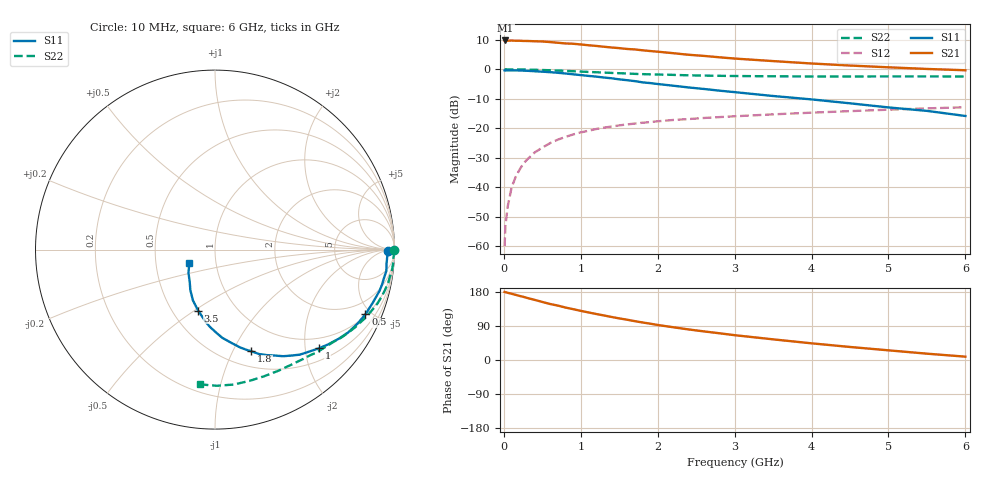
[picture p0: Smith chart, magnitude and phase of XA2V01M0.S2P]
! SIEMENS Discrete & RF Semiconductors
! BFY180
! Si NPN RF Bipolar Junction Transistor in MICRO-X
! VCE = 2 V  IC = 1 mA
! Common Emitter S-Parameters:  May  1997
# GHz  S  MA  R  50
!  f  S11  S21  S12  S22
! GHz  MAG  ANG  MAG  ANG  MAG  ANG  MAG  ANG
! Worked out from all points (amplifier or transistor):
!   36 points, 10 MHz to 6 GHz, reference 50 ohm
!   highest |S21| = 9.8 dB at 20 MHz (marker M1)
!   |S21| within 3 dB of that: start of sweep to 1.673 GHz
!   unconditionally stable (mu >= 1): 3.663 GHz to end of sweep
!   at 250 MHz: K = 0.08, MSG = 20.9 dB, |S12| = -32.1 dB
!   at 1.4 GHz: K = 0.53, MSG = 13.4 dB, |S12| = -19.4 dB
!   at 6 GHz: K = 1.07, MAG = 4.6 dB, |S12| = -12.9 dB
!   S11 on the Smith chart (normalised r, x): 10 MHz: 50, -9; 500 MHz: 1.07, -4.61; 1 GHz: 0.76, -2.29; 1.8 GHz: 0.67, -1.19; 3.5 GHz: 0.67, -0.52; 6 GHz: 0.74, -0.11
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0.01  0.9616 -0.4  3.072 179.6  0.001 86.6  0.9972 -0.2
0.02  0.9574 -0.7  3.089 178.9  0.0022 86.3  0.9999 -0.5
0.05  0.9605 -2.2  3.064 177.4  0.0047 87.1  0.9969 -1.4
0.1  0.9589 -4.8  3.083 174.8  0.0098 87.9  0.995 -2.8
0.15  0.962 -7.1  3.054 172.2  0.0146 85.2  0.996 -4.1
0.25  0.951 -11.7  3.032 166.9  0.0248 82.7  0.9928 -6.8
0.4  0.9277 -18.6  2.995 158.7  0.0388 77.6  0.9829 -10.7
0.5  0.9123 -23.3  2.97 153.2  0.047 73.9  0.9736 -13.4
0.6  0.8953 -27.4  2.902 147.8  0.0558 71.1  0.9643 -15.8
0.9  0.8229 -39.9  2.717 134.2  0.0785 62.4  0.9289 -22.8
1  0.7987 -43.5  2.642 129.7  0.0851 59.8  0.9165 -25.0
1.1  0.774 -47.2  2.561 125.5  0.0907 57.6  0.9032 -27.0
1.2  0.7522 -51.1  2.495 121.4  0.0971 55.2  0.8924 -29.1
1.5  0.676 -60.8  2.289 109.8  0.112 49.4  0.8598 -34.5
1.8  0.6021 -70.3  2.105 99.1  0.1241 44.9  0.8298 -39.3
2.2  0.5279 -80.0  1.88 86.5  0.1383 39.3  0.8053 -45.4
2.4  0.493 -85.3  1.767 80.7  0.1433 37.2  0.7916 -48.1
2.8  0.435 -93.2  1.601 70.6  0.1547 33.5  0.7761 -53.4
3.5  0.3529 -105.4  1.38 54.5  0.1723 27.4  0.7619 -62.3
4.5  0.2651 -121.2  1.16 34.4  0.1954 19.8  0.7563 -75.3
5.5  0.1974 -138.5  1.015 16.7  0.2176 11.9  0.7588 -89.2
6  0.1617 -152.4  0.964 8.8  0.2273 7.7  0.7554 -96.2
